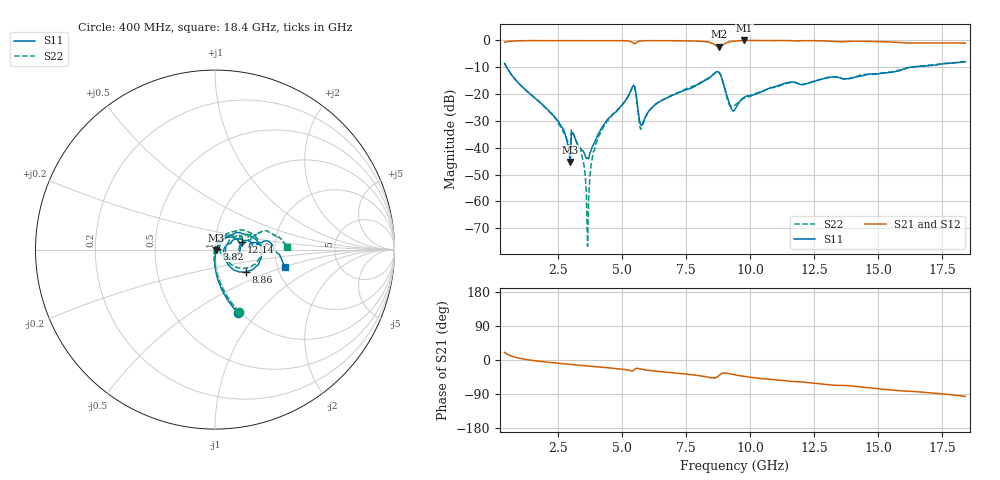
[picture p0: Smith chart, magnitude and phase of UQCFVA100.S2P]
!  Part Number  UQCFVA100  Mounting Orientation: Horizontal
!  Description: Ultra Low ESR Microwave capacitors
!  Application: Coupling, Bypass, Tuning, DC Block
!  Filters, Matching
# GHZ S DB R 50
! Freq  |S11|  S11 Ph  |S21|  S21 Ph  |S12|  S12 Ph  |S22|  S22 Ph
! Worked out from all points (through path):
!   401 points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, 400 MHz to 18.4 GHz, reference 50 ohm
!   highest |S21| = 0.00 dB at 9.76 GHz (marker M1); lowest = -2.4 dB at 8.77 GHz (marker M2)
!   group delay of S21, straight-line fit = 15.2 ps
!   lowest |S11| = -45.4 dB at 2.965 GHz (marker M3), VSWR 1.01, Z = 50.4 - j0.407 ohm
!   |S11| at or under -10 dB: 480.6 MHz to 16.24 GHz (15.76 GHz wide, 189 % of centre)
!   |S22| runs from -76.7 to -7.9 dB; largest |S21 - S12| = 0.0059
!   S11 on the Smith chart (normalised r, x): 400 MHz: 0.97, -0.79; 3.82 GHz: 1.02, +0.01; 8.86 GHz: 1.36, -0.36; 12.14 GHz: 1.34, +0.11; 18.4 GHz: 2.18, -0.51
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0.4  -8.57 -70.1  -0.67 20.1  -0.70 20.1  -8.59 -69.0
2.425  -29.31 -87.3  -0.04 -8.2  -0.07 -8.1  -29.48 -101.9
2.965  -45.35 -48.4  -0.03 -11.6  -0.06 -11.5  -39.93 -114.5
3.1  -35.22 -84.5  -0.03 -12.6  -0.06 -12.5  -34.93 -103.3
3.415  -40.92 -49.9  -0.05 -14.4  -0.07 -14.3  -42.88 -100.3
3.64  -43.76 -6.9  -0.05 -15.7  -0.07 -15.6  -76.71 25.8
3.73  -42.02 20.5  -0.05 -16.2  -0.07 -16.1  -50.87 89.2
3.82  -39.73 33.2  -0.05 -16.8  -0.07 -16.6  -44.24 88.8
4.27  -31.47 55.0  -0.06 -19.5  -0.08 -19.3  -32.09 77.1
5.395  -17.27 23.9  -0.75 -28.7  -0.76 -28.5  -17.44 30.1
5.755  -31.62 13.0  -0.15 -24.6  -0.16 -24.4  -32.41 25.6
6.43  -22.99 50.3  -0.08 -30.2  -0.08 -30.1  -22.90 58.0
8.32  -14.48 26.1  -0.52 -44.9  -0.50 -44.6  -14.22 33.5
8.77  -11.87 -19.1  -2.35 -41.3  -2.32 -41.0  -11.90 -10.5
8.86  -13.42 -36.1  -2.07 -36.3  -2.04 -36.1  -13.36 -27.8
9.175  -23.10 -39.5  -0.52 -36.3  -0.50 -36.1  -24.00 -24.1
9.4  -25.69 6.5  -0.22 -39.6  -0.19 -39.3  -24.15 11.3
9.76  -21.17 22.8  0.00 -43.2  -0.01 -42.9  -21.59 27.3
12.145  -16.24 15.4  -0.07 -58.8  -0.05 -58.8  -16.23 26.2
12.415  -15.49 17.1  -0.06 -60.8  -0.04 -60.8  -15.41 28.0
15.43  -11.99 7.7  -0.56 -78.7  -0.53 -78.9  -11.82 20.8
18.4  -7.96 -14.2  -1.01 -96.1  -0.97 -96.4  -7.88 2.0
